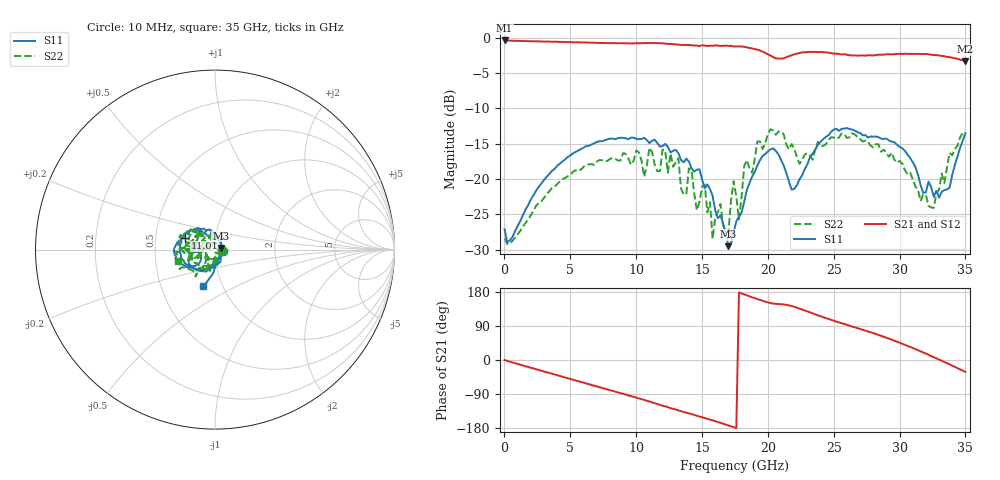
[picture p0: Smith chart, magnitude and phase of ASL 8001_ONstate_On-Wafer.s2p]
!ASL 8001 Wideband SPST Switch
!ON State On-Wafer S-parameter data from 10MHz-35 GHz
!Agilent Technologies,E8363B,MY43030569,A.06.01.05
!Agilent E8363B: A.06.01.05
!Date: Thursday, August 10, 2006 16:54:05
!Correction: S11(Full 2 Port(1,2)) S21(Full 2 Port(1,2)) S12(Full 2 Port(1,2)) S22(Full 2 Port(1,2))
!S2P File: Measurements: S11, S21, S12, S22:
# Hz S  dB  R 50
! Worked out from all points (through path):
!   176 points, 10 MHz to 35 GHz, reference 50 ohm
!   highest |S21| = -0.38 dB at 10 MHz (marker M1); lowest = -3.3 dB at 35 GHz (marker M2)
!   group delay of S21, straight-line fit = 29.8 ps
!   lowest |S11| = -29.5 dB at 17.01 GHz (marker M3), VSWR 1.07, Z = 53.3 + j0.912 ohm
!   |S11| at or under -10 dB: start of sweep to end of sweep
!   |S22| runs from -29.2 to -12.9 dB; largest |S21 - S12| = 0.0087
!   S11 on the Smith chart (normalised r, x): 10 MHz: 1.09, -0.02; 11.01 GHz: 0.71, +0.10; 35 GHz: 0.81, -0.34
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1e7  -27.10 -9.0  -0.38 -0.2  -0.34 0.2  -28.40 -5.4
6.0085e9  -15.56 -143.3  -0.66 -60.0  -0.67 -59.9  -18.25 -135.1
1.00075e10  -14.29 169.3  -0.75 -99.1  -0.77 -99.1  -15.94 179.1
1.060735e10  -14.16 162.7  -0.74 -105.4  -0.75 -105.3  -19.66 174.3
1.100725e10  -14.91 158.5  -0.72 -109.5  -0.73 -109.4  -15.57 165.5
1.180705e10  -15.40 149.2  -0.78 -118.2  -0.79 -118.1  -18.85 144.6
1.32067e10  -16.33 127.7  -0.98 -132.9  -0.99 -132.9  -17.05 165.6
1.36066e10  -17.64 128.9  -1.02 -137.3  -1.02 -137.3  -22.16 158.7
1.40065e10  -17.52 118.6  -1.02 -140.8  -1.04 -140.7  -18.48 131.8
1.48063e10  -18.61 105.0  -1.16 -149.3  -1.18 -149.3  -23.25 76.8
1.700575e10  -29.50 14.8  -1.14 -172.6  -1.15 -172.4  -27.48 168.2
1.740565e10  -27.51 -21.0  -1.22 -177.1  -1.23 -177.0  -20.30 -109.7
1.76056e10  -25.98 -45.0  -1.22 -179.7  -1.23 -179.6  -22.47 -85.5
1.780555e10  -25.28 -64.4  -1.21 177.9  -1.24 177.9  -25.69 -91.2
1.820545e10  -23.21 -77.5  -1.27 173.2  -1.29 173.3  -18.18 -122.6
2.020495e10  -15.80 -145.0  -2.51 150.2  -2.52 150.2  -12.93 -151.0
2.180455e10  -21.49 -164.8  -2.48 142.5  -2.49 142.5  -15.03 174.1
2.340415e10  -16.40 -142.6  -2.00 123.1  -1.99 123.0  -17.26 -176.2
2.56036e10  -12.88 -173.2  -2.36 97.0  -2.33 96.9  -13.54 172.8
2.92027e10  -14.55 150.3  -2.33 56.4  -2.34 56.1  -16.85 139.2
3.260185e10  -22.49 85.0  -2.44 7.5  -2.45 7.5  -24.07 -175.8
3.500125e10  -13.50 -108.0  -3.32 -31.4  -3.28 -31.1  -13.42 -163.2
